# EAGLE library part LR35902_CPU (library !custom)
Sharp LR35902 CPU Z80/8080 Hybrid used in the DMG-01 The origional spec cannot be found, so assumptions are made. This thin quad flat pack (TQFP) uses a common spacing of 0.8mm between the pins. When compaired to a scaled photo, the solder pads match very closely.
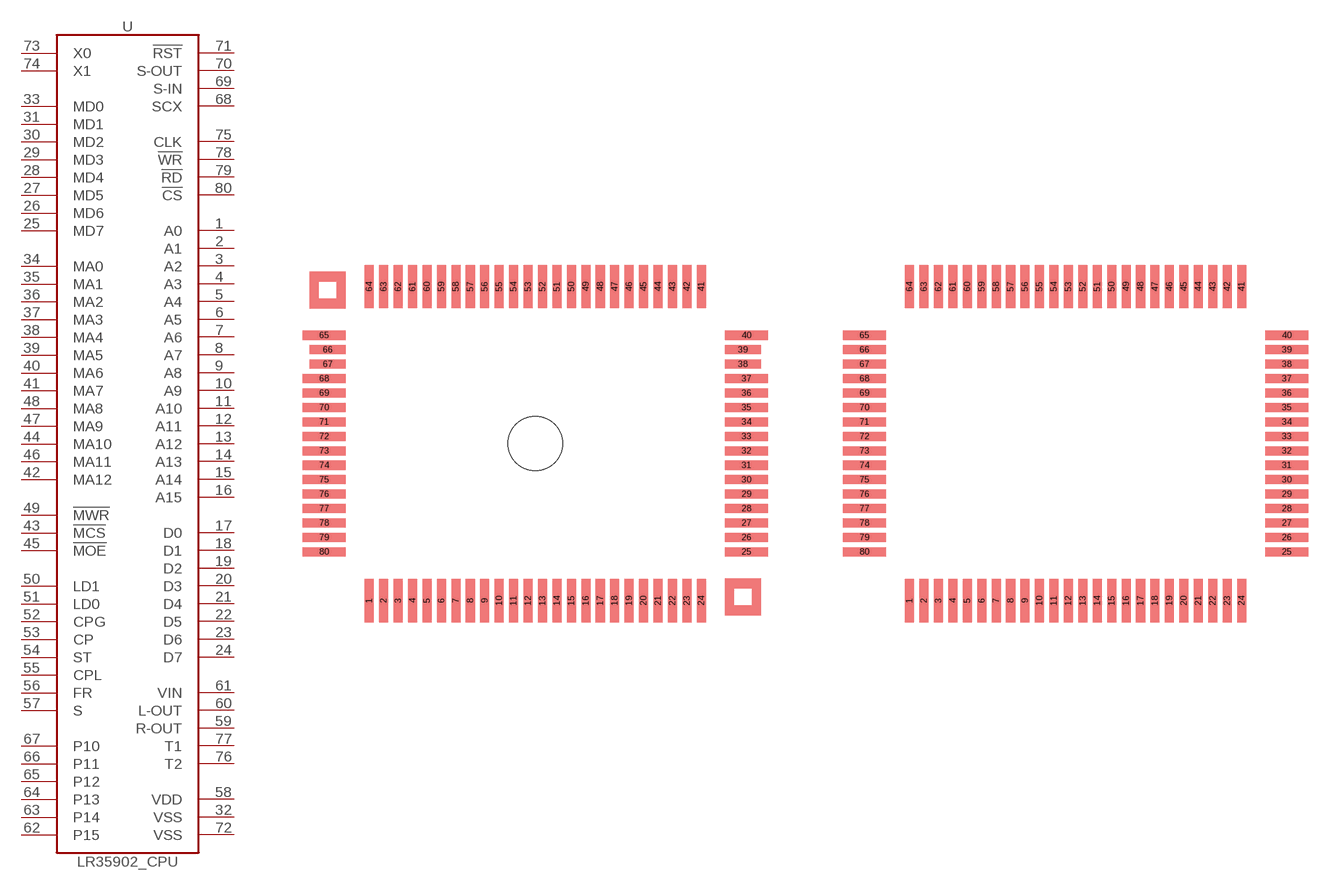
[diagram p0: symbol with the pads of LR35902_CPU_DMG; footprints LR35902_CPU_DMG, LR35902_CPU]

Designator prefix -

## LR35902_CPU_DMG  [LR35902_CPU_DMG]
1  A0  pas
2  A1  pas
3  A2  pas
4  A3  pas
5  A4  pas
6  A5  pas
7  A6  pas
8  A7  pas
9  A8  pas
10  A9  pas
11  A10  pas
12  A11  pas
13  A12  pas
14  A13  pas
15  A14  pas
16  A15  pas
17  D0  pas
18  D1  pas
19  D2  pas
20  D3  pas
21  D4  pas
22  D5  pas
23  D6  pas
24  D7  pas
25  MD7  pas
26  MD6  pas
27  MD5  pas
28  MD4  pas
29  MD3  pas
30  MD2  pas
31  MD1  pas
32  VSS  pas
33  MD0  pas
34  MA0  pas
35  MA1  pas
36  MA2  pas
37  MA3  pas
38  MA4  pas
39  MA5  pas
40  MA6  pas
41  MA7  pas
42  MA12  pas
43  !MCS  pas
44  MA10  pas
45  !MOE  pas
46  MA11  pas
47  MA9  pas
48  MA8  pas
49  !MWR  pas
50  LD1  pas
51  LD0  pas
52  CPG  pas
53  CP  pas
54  ST  pas
55  CPL  pas
56  FR  pas
57  S  pas
58  VDD  pas
59  R-OUT  pas
60  L-OUT  pas
61  VIN  pas
62  P15  pas
63  P14  pas
64  P13  pas
65  P12  pas
66  P11  pas
67  P10  pas
68  SCX  pas
69  S-IN  pas
70  S-OUT  pas
71  !RST  pas
72  VSS  pas
73  X0  pas
74  X1  pas
75  CLK  pas
76  T2  pas
77  T1  pas
78  !WR  pas
79  !RD  pas
80  !CS  pas

## LR35902_CPU  [LR35902_CPU]
Pads as for LR35902_CPU_DMG

## Footprint LR35902_CPU_DMG (pad centres in mm)
smd 0.5 x 2.4: 1 -9.2,-8.7; 2 -8.4,-8.7; 3 -7.6,-8.7; 4 -6.8,-8.7; 5 -6,-8.7; 6 -5.2,-8.7; 7 -4.4,-8.7; 8 -3.6,-8.7; 9 -2.8,-8.7; 10 -2,-8.7; 11 -1.2,-8.7; 12 -0.4,-8.7; 13 0.4,-8.7; 14 1.2,-8.7; 15 2,-8.7; 16 2.8,-8.7; 17 3.6,-8.7; 18 4.4,-8.7; 19 5.2,-8.7; 20 6,-8.7; 21 6.8,-8.7; 22 7.6,-8.7; 23 8.4,-8.7; 24 9.2,-8.7; 41 9.2,8.7; 42 8.4,8.7; 43 7.6,8.7; 44 6.8,8.7; 45 6,8.7; 46 5.2,8.7; 47 4.4,8.7; 48 3.6,8.7; 49 2.8,8.7; 50 2,8.7; 51 1.2,8.7; 52 0.4,8.7; 53 -0.4,8.7; 54 -1.2,8.7; 55 -2,8.7; 56 -2.8,8.7; 57 -3.6,8.7; 58 -4.4,8.7; 59 -5.2,8.7; 60 -6,8.7; 61 -6.8,8.7; 62 -7.6,8.7; 63 -8.4,8.7; 64 -9.2,8.7
smd 2.4 x 0.5: 25 11.7,-6; 26 11.7,-5.2; 27 11.7,-4.4; 28 11.7,-3.6; 29 11.7,-2.8; 30 11.7,-2; 31 11.7,-1.2; 32 11.7,-0.4; 33 11.7,0.4; 34 11.7,1.2; 35 11.7,2; 36 11.7,2.8; 37 11.7,3.6; 40 11.7,6; 65 -11.7,6; 68 -11.7,3.6; 69 -11.7,2.8; 70 -11.7,2; 71 -11.7,1.2; 72 -11.7,0.4; 73 -11.7,-0.4; 74 -11.7,-1.2; 75 -11.7,-2; 76 -11.7,-2.8; 77 -11.7,-3.6; 78 -11.7,-4.4; 79 -11.7,-5.2; 80 -11.7,-6
smd 2 x 0.5: 38 11.5,4.4; 39 11.5,5.2; 66 -11.5,5.2; 67 -11.5,4.4
hole 3 at 0,0

## Footprint LR35902_CPU (pad centres in mm)
smd 0.5 x 2.4: 1 -9.2,-8.7; 2 -8.4,-8.7; 3 -7.6,-8.7; 4 -6.8,-8.7; 5 -6,-8.7; 6 -5.2,-8.7; 7 -4.4,-8.7; 8 -3.6,-8.7; 9 -2.8,-8.7; 10 -2,-8.7; 11 -1.2,-8.7; 12 -0.4,-8.7; 13 0.4,-8.7; 14 1.2,-8.7; 15 2,-8.7; 16 2.8,-8.7; 17 3.6,-8.7; 18 4.4,-8.7; 19 5.2,-8.7; 20 6,-8.7; 21 6.8,-8.7; 22 7.6,-8.7; 23 8.4,-8.7; 24 9.2,-8.7; 41 9.2,8.7; 42 8.4,8.7; 43 7.6,8.7; 44 6.8,8.7; 45 6,8.7; 46 5.2,8.7; 47 4.4,8.7; 48 3.6,8.7; 49 2.8,8.7; 50 2,8.7; 51 1.2,8.7; 52 0.4,8.7; 53 -0.4,8.7; 54 -1.2,8.7; 55 -2,8.7; 56 -2.8,8.7; 57 -3.6,8.7; 58 -4.4,8.7; 59 -5.2,8.7; 60 -6,8.7; 61 -6.8,8.7; 62 -7.6,8.7; 63 -8.4,8.7; 64 -9.2,8.7
smd 2.4 x 0.5: 25 11.7,-6; 26 11.7,-5.2; 27 11.7,-4.4; 28 11.7,-3.6; 29 11.7,-2.8; 30 11.7,-2; 31 11.7,-1.2; 32 11.7,-0.4; 33 11.7,0.4; 34 11.7,1.2; 35 11.7,2; 36 11.7,2.8; 37 11.7,3.6; 38 11.7,4.4; 39 11.7,5.2; 40 11.7,6; 65 -11.7,6; 66 -11.7,5.2; 67 -11.7,4.4; 68 -11.7,3.6; 69 -11.7,2.8; 70 -11.7,2; 71 -11.7,1.2; 72 -11.7,0.4; 73 -11.7,-0.4; 74 -11.7,-1.2; 75 -11.7,-2; 76 -11.7,-2.8; 77 -11.7,-3.6; 78 -11.7,-4.4; 79 -11.7,-5.2; 80 -11.7,-6

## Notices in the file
If you are not the copyright holder, your usage of applicable works is licensed under a Creative Commons Attribution-NonCommercial-NoDerivatives 4.0 (or later) International License.
